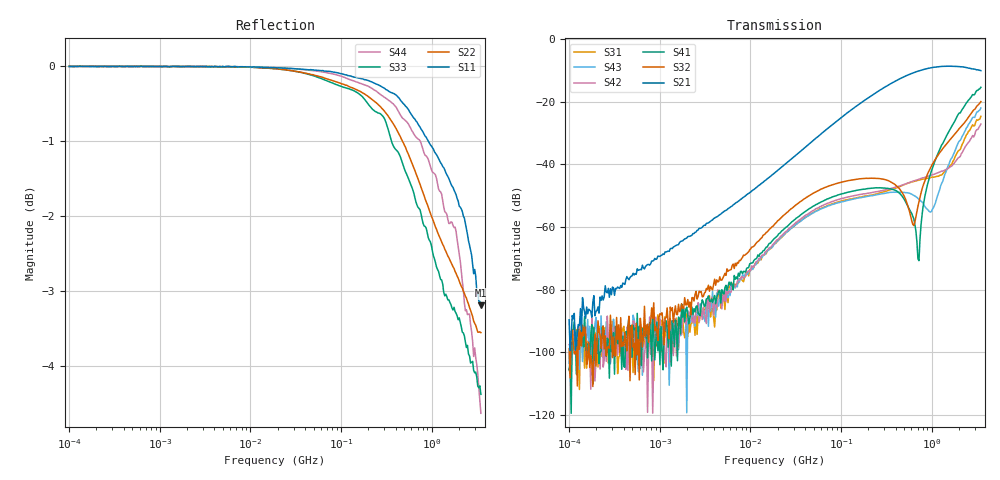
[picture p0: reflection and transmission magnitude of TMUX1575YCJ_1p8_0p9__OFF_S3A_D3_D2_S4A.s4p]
!Keysight Technologies,E5080A,MY55200740,A.12.60.03
!Date: Tuesday, July 21, 2020 11:53:38
!Correction: S11(Full 4 Port(1,2,3,4))
!S12(Full 4 Port(1,2,3,4))
!S13(Full 4 Port(1,2,3,4))
!S14(Full 4 Port(1,2,3,4))
!S21(Full 4 Port(1,2,3,4))
!S22(Full 4 Port(1,2,3,4))
!S23(Full 4 Port(1,2,3,4))
!S24(Full 4 Port(1,2,3,4))
!S31(Full 4 Port(1,2,3,4))
!S32(Full 4 Port(1,2,3,4))
!S33(Full 4 Port(1,2,3,4))
!S34(Full 4 Port(1,2,3,4))
!S41(Full 4 Port(1,2,3,4))
!S42(Full 4 Port(1,2,3,4))
!S43(Full 4 Port(1,2,3,4))
!S44(Full 4 Port(1,2,3,4))
!S4P File: Measurements: <S11,S12,S13,S14>,
!<S21,S22,S23,S24>,
!<S31,S32,S33,S34>,
!<S41,S42,S43,S44>:Log Frequency Sweep
# Hz S  dB  R 50
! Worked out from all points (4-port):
!   400 points, 100 kHz to 3.5 GHz, reference 50 ohm
!   strongest paths, dB at 100 kHz, 1.377 MHz, 18.96 MHz, 261 MHz, 3.5 GHz:
!     S21: -89.7, -66.9, -42.5, -16.5, -10.0
!     S32: -99.0, -85.8, -58.8, -44.5, -19.9
!     S41: -105.7, -90.0, -63.4, -47.5, -15.4
!     S42: -97.6, -95.3, -64.7, -48.6, -27.1
!     S43: -103.6, -94.7, -65.1, -49.6, -22.0
!     S31: -105.4, -95.5, -65.3, -49.3, -24.6
!   lowest |S11| = -3.2 dB at 3.5 GHz (marker M1), VSWR 5.51, Z = 11.8 - j26.9 ohm
!   |S11| at or under -10 dB: nowhere
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100000  0.00 -0.0  -97.10 55.4  -106.91 -14.7  -96.65 -101.2
        -89.68 89.5  0.00 -0.0  -95.22 82.8  -97.53 -146.7
        -105.42 -155.4  -98.98 -144.8  0.00 -0.0  -100.14 -88.8
        -105.70 42.4  -97.60 75.2  -103.60 72.1  0.00 -0.0
6468358  -0.00 -0.6  -53.01 96.8  -78.99 128.5  -78.26 111.9
         -52.93 96.6  -0.00 -0.9  -72.27 115.9  -79.05 123.2
         -77.91 114.7  -71.87 109.4  -0.00 -1.0  -79.24 116.2
         -80.12 114.8  -79.30 113.8  -79.85 105.2  -0.00 -0.6
2.349838e8  -0.22 -16.3  -17.36 75.0  -49.59 34.5  -47.55 35.6
            -17.36 75.0  -0.46 -26.8  -44.49 23.9  -48.83 31.4
            -49.60 34.4  -44.44 23.7  -0.59 -28.8  -49.89 31.9
            -47.51 35.5  -48.83 31.3  -49.85 32.0  -0.32 -18.2
5.026996e8  -0.51 -32.7  -11.93 51.6  -46.45 24.8  -51.29 23.5
            -11.92 51.7  -1.05 -51.8  -50.38 12.4  -46.40 22.7
            -46.45 24.8  -50.37 12.4  -1.37 -55.9  -48.97 15.4
            -51.33 23.6  -46.39 22.9  -48.98 15.8  -0.71 -36.5
7.256873e8  -0.79 -44.6  -10.11 37.6  -45.06 8.5  -70.25 155.5
            -10.11 37.5  -1.53 -67.7  -51.92 134.2  -44.76 11.8
            -45.04 8.6  -51.93 134.5  -1.89 -72.8  -51.17 -5.9
            -70.77 155.6  -44.74 11.7  -51.19 -5.7  -0.97 -48.7
1.047588e9  -1.10 -59.0  -9.00 22.6  -44.13 -25.5  -40.30 -171.2
            -8.99 22.7  -2.06 -84.2  -39.41 141.5  -43.26 -9.9
            -44.09 -25.5  -39.41 141.4  -2.53 -90.4  -53.68 -94.9
            -40.27 -171.4  -43.25 -9.9  -53.82 -95.2  -1.42 -63.6
3.5e9  -3.19 -121.3  -10.04 -20.4  -24.61 154.8  -15.34 126.8
       -10.03 -20.5  -3.55 -131.1  -19.89 135.1  -27.09 172.0
       -24.63 154.8  -19.94 135.0  -4.37 -142.3  -21.99 135.4
       -15.36 126.7  -27.12 172.0  -21.98 135.6  -4.63 -125.2
